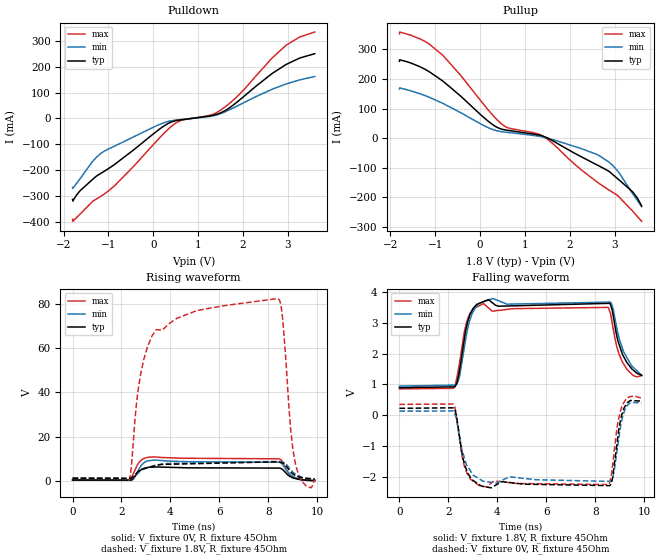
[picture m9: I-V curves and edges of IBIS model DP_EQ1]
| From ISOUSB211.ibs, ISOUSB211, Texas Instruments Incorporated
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[Model]   DP_EQ1
Model_type   Output
Polarity   Non-Inverting
Vmeas = 0.2
Vref = 0
Cref = 15pF
Rref = 45
|   typ   min   max
C_comp   5pF   3pF   8pF
[Voltage Range]   1.8   1.71   1.89
[Temperature Range]   27   150   -40
[Pullup Reference]   1.8   1.71   1.89
[Pulldown Reference]   0   0   0
[Power Clamp Reference]   1.8   1.71   1.89
[GND Clamp Reference]   0   0   0
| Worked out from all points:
|   slope of the pulldown table from 0 to 0.27 V, typ, clamps not added: 7.95 ohm
|   slope of the pullup table from 0 to 0.27 V, typ, clamps not added: 7.94 ohm
|   falling waveform, V_fixture 1.8V, R_fixture 45Ohm: 20-80 % time 97.9ps typ, 103ps min, 94.6ps max; typ from 0.895 V to 1.3 V
|   rising waveform, V_fixture 0V, R_fixture 45Ohm: 20-80 % time 223ps typ, 148ps min, 108ps max; typ from 0.46 V to 0.225 V
|   rising waveform, V_fixture 1.8V, R_fixture 45Ohm: 20-80 % time 296ps typ, 197ps min, 52.8ps max; typ from 1.3 V to 0.895 V
|   falling waveform, V_fixture 0V, R_fixture 45Ohm: 20-80 % time 112ps typ, 126ps min, 92.4ps max; typ from 0.225 V to 0.46 V
[Pulldown]
|   Voltage   I(typ)   I(min)   I(max)
-1.8V     -312.3mA   -266.2mA   -388.8mA
-1.795V   -319mA     -269.8mA   -396.8mA
-1.633V   -278.9mA   -232.8mA   -369.2mA
-1.179V   -212.7mA   -136mA     -301.6mA
-865.8mV  -177.8mA   -106.8mA   -260mA
73.8mV    -49.63mA   -27.98mA   -87.09mA
538.2mV   -7.266mA   -5.626mA   -13.71mA
1.294V    10.85mA    9.019mA    13.98mA
1.521V    23.18mA    20.15mA    34.45mA
1.899V    67.71mA    50.57mA    89.7mA
2.947V    206.8mA    132.3mA    280.4mA
3.6V      250.2mA    161.9mA    333.6mA
[Pullup]
|   Voltage   I(typ)   I(min)   I(max)
-1.8V     259.8mA    166.3mA    352.1mA
-1.795V   264.8mA    169.7mA    358.5mA
-1.325V   240.1mA    149.1mA    334.3mA
-849.6mV  194.9mA    118.9mA    282mA
381.6mV   36.3mA     24.84mA    61.51mA
613.8mV   26.64mA    19.55mA    35.63mA
1.402V    6.733mA    3.773mA    6.537mA
2.612V    -90.76mA   -55.24mA   -148.5mA
2.876V    -112.3mA   -81.28mA   -175.5mA
3.065V    -136.9mA   -110.7mA   -193.6mA
3.4V      -181.3mA   -187.3mA   -246.2mA
3.6V      -228.6mA   -231.2mA   -280.5mA
[Ramp]
R_load = 45
|   typ   min   max
dV/dt_r   0.140808/7.42864e-09   0.160407/7.53653e-09   0.120509/5.34817e-09
dV/dt_f   0.243789/8.82719e-11   0.210518/9.29553e-11   0.256824/8.57593e-11
[Falling Waveform]
V_fixture = 1.8V
V_fixture_min = 1.71V
V_fixture_max = 1.89V
R_fixture = 45Ohm
C_fixture = 0F
|   Time   V(typ)   V(min)   V(max)
0s        895mV      947.6mV    856.5mV
2.268ns   924mV      980.3mV    973.5mV
2.462ns   1.495V     1.286V     1.731V
2.806ns   3.083V     2.873V     3.172V
3.111ns   3.565V     3.507V     3.503V
3.63ns    3.76V      3.745V     3.5V
8.619ns   3.616V     3.682V     3.326V
8.881ns   2.595V     2.847V     2.238V
9.11ns    1.997V     2.189V     1.738V
9.9ns     1.301V     1.298V     1.285V
[Rising Waveform]
V_fixture = 0V
V_fixture_min = 0V
V_fixture_max = 0V
R_fixture = 45Ohm
C_fixture = 0F
|   Time   V(typ)   V(min)   V(max)
0s        459.5mV    400.3mV    553.4mV
2.307ns   414.8mV    339.5mV    501.5mV
2.503ns   1.501V     1.218V     3.844V
2.784ns   4.953V     6.645V     9.223V
2.985ns   5.91V      8.719V     10.47V
3.319ns   6.322V     9.426V     10.9V
8.436ns   5.86V      8.487V     10.05V
8.817ns   2.619V     3.927V     3.694V
8.998ns   1.483V     2.205V     1.873V
9.9ns     224.9mV    133mV      352.5mV
[Rising Waveform]
V_fixture = 1.8V
V_fixture_min = 1.71V
V_fixture_max = 1.89V
R_fixture = 45Ohm
C_fixture = 0F
|   Time   V(typ)   V(min)   V(max)
0s        1.301V     1.298V     1.285V
2.312ns   1.204V     1.188V     476.2mV
2.771ns   4.914V     4.49V      47.47V
3.414ns   6.973V     7.205V     68.24V
8.363ns   8.682V     8.855V     82.32V
8.563ns   8.273V     8.572V     75.67V
8.902ns   4.35V      5.332V     24.96V
9.102ns   2.52V      3.2V       8.293V
9.535ns   1.196V     1.337V     -2.067V
9.9ns     895mV      947.6mV    856.5mV
[Falling Waveform]
|Gnd
V_fixture = 0V
V_fixture_min = 0V
V_fixture_max = 0V
R_fixture = 45Ohm
C_fixture = 0F
|   Time   V(typ)   V(min)   V(max)
0s        224.9mV    133mV      352.5mV
2.207ns   240.6mV    138.3mV    365.1mV
2.663ns   -1.592V    -1.412V    -1.681V
3.258ns   -2.258V    -2.07V     -2.29V
8.523ns   -2.291V    -2.153V    -2.257V
8.755ns   -1.773V    -1.918V    -1.336V
8.924ns   -737.4mV   -995.1mV   -268.2mV
9.102ns   43.16mV    -129.5mV   316.4mV
9.451ns   477.9mV    417.4mV    606.9mV
9.9ns     459.5mV    400.3mV    553.4mV
